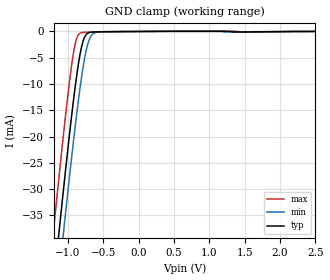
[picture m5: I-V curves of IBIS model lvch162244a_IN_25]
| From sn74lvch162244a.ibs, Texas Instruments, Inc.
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[Model]   lvch162244a_IN_25
Model_type  Input
Vinl=0.7
Vinh=1.7
| variable   typ   min   max
C_comp   3.32pF   2.57pF   4.47pF
[Temperature Range]   40   100   -40
| Ambient temperature   25   85   -40
[Voltage range]   2.5   2.3   2.7
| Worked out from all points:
|   GND clamp passes 1 mA (typ) near -0.76 V on its own axis
[GND Clamp]
| lvch162244a_IN_25
|   Voltage   I(typ)   I(min)   I(max)
-5.5V     -656.7mA   -663.5mA   -648.5mA
-1.205V   -48.51mA   -56.74mA   -37.96mA
-1.13V    -38.63mA   -46.87mA   -28.07mA
-1.07V    -30.91mA   -39.11mA   -20.4mA
-1.055V   -29mA      -37.2mA    -18.53mA
-965mV    -18mA      -25.99mA   -8.116mA
-885mV    -9.237mA   -16.65mA   -1.681mA
-825mV    -4.045mA   -10.35mA   -313.2uA
-775mV    -1.402mA   -5.908mA   -175.3uA
-710mV    -271.2uA   -1.984mA   -144.6uA
-640mV    -99.44uA   -393.7uA   -125.6uA
2.5V      7.214pA    38.93nA    -770.4pA
